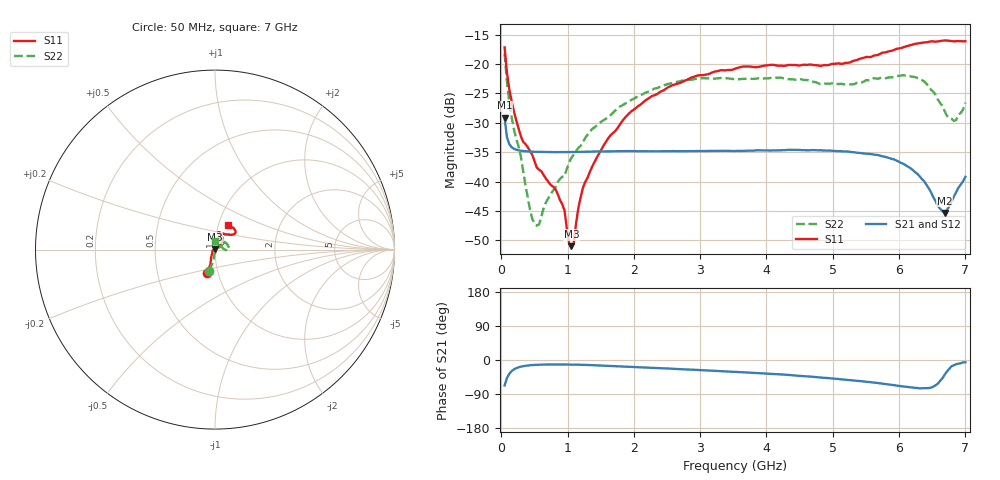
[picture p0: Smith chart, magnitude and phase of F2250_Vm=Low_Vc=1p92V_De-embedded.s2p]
! Integrated Device Technology
! Corporate Headquarters
! 6024 Silver Creek Valley Road
! San Jose, CA 95138  USA
! Phone:  1-408-284-8200
! Toll Free:  1-800-223-1366
! Webpage:  http://www.idt.com/
! Timing and RF Division
! 515 Groton Road, Suite 102
! Westford, MA 01886-6024
! Device:  F2250
! Description: Voltage Variable RF Attenuator
! Frequency:  50.0 -  6000.00 MHz
! Package:  3x3 mm Thin QFN Plastic Package: 16 pin
! Ports:  2 RF, 3 DC
!  Pin  1  = GND
!  Pin  2  = NC
!  Pin  3  = RF1  = Port 1
!  Pin  4  = NC
!  Pin  5  = GND
!  Pin  6  = GND
!  Pin  7  = GND
!  Pin  8  = GND
!  Pin  9  = NC
!  Pin 10  = RF2  = Port 2
!  Pin 11  = NC
!  Pin 12  = GND
!  Pin 13  = GND
!  Pin 14  = VCNTRL
!  Pin 15  = VDD
!  Pin 16  = VMODE
! Vcntrl:  1.920 Volts
! Vmode:  +0.000 Volts
! Vdd:  +3.30  Volts
! Current:  1.182 mA
! Data:  The device was measured on a the F2250 evaluation board which has
!  individual transmission lines to the RF pins.  Data was collected
!  using a calibrated network analyzer.  The evaluation board was
!  de-embedded using a TRL calibration technique.
!  The reference plane is the edge of the package pin.
! Misc:  SN 10
!  Action Tracker AT0258
! Date Measured:  2014-11-26
! Date:  2015-10-15  MJV
! Note:
!  Integrated Device Technology supplies this data as a sample of measured
!  data at the package pin for this product.  Your particular data for this
!  product may vary.
!  Data was taken at 25 degrees C.
!  Integrated Device Technology reserves the right to change this data at anytime.
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# GHz S dB R 50
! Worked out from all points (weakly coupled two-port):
!   201 points, 50 MHz to 7 GHz, reference 50 ohm
!   highest |S21| = -29.15 dB at 50 MHz (marker M1); lowest = -45.4 dB at 6.687 GHz (marker M2)
!   lowest |S11| = -51.0 dB at 1.058 GHz (marker M3), VSWR 1.01, Z = 49.9 + j0.242 ohm
!   |S11| at or under -10 dB: start of sweep to end of sweep
!   |S22| runs from -47.5 to -18.2 dB; largest |S21 - S12| = 5.6e-05
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0.05  -17.17 -108.5  -29.15 -67.0  -29.15 -67.0  -18.18 -106.3
0.1195  -24.20 -111.6  -33.61 -36.6  -33.60 -36.6  -26.40 -97.9
0.22375  -29.52 -121.9  -34.57 -21.8  -34.57 -21.8  -32.64 -94.5
0.50175  -36.56 -149.4  -34.93 -13.0  -34.93 -13.0  -47.19 -36.6
0.57125  -37.99 -160.1  -34.95 -12.4  -34.95 -12.4  -47.25 -9.5
0.6755  -39.52 -163.2  -34.97 -11.9  -34.97 -11.9  -43.49 13.8
0.91875  -43.83 158.0  -34.99 -11.8  -34.99 -11.8  -39.17 25.9
0.9535  -44.90 169.6  -34.99 -11.9  -34.99 -11.9  -39.10 32.7
1.023  -50.51 143.1  -34.98 -12.0  -34.98 -12.0  -36.68 32.1
1.05775  -50.98 120.6  -34.97 -12.1  -34.98 -12.1  -35.96 32.7
1.0925  -50.52 87.6  -34.97 -12.2  -34.97 -12.2  -35.43 31.5
1.162  -44.53 55.7  -34.95 -12.4  -34.95 -12.4  -34.28 27.8
1.2315  -41.05 43.2  -34.93 -12.7  -34.93 -12.7  -33.29 25.9
1.6485  -32.10 41.6  -34.86 -15.5  -34.86 -15.5  -28.69 32.8
2.37825  -24.87 47.2  -34.83 -21.5  -34.84 -21.5  -23.97 39.3
3.525  -20.81 72.4  -34.80 -31.2  -34.80 -31.2  -22.59 64.7
4.7065  -20.18 72.3  -34.64 -44.5  -34.63 -44.5  -23.03 66.2
5.85325  -17.82 40.4  -36.01 -64.8  -36.01 -64.9  -22.26 12.9
6.33975  -16.40 40.9  -39.51 -74.6  -39.50 -74.7  -22.69 -1.3
6.68725  -15.99 48.8  -45.35 -38.7  -45.33 -38.5  -28.01 18.9
6.82625  -16.14 53.6  -42.54 -13.7  -42.48 -13.7  -29.68 52.0
7  -16.13 63.2  -39.19 -6.0  -39.15 -6.1  -26.57 90.9
